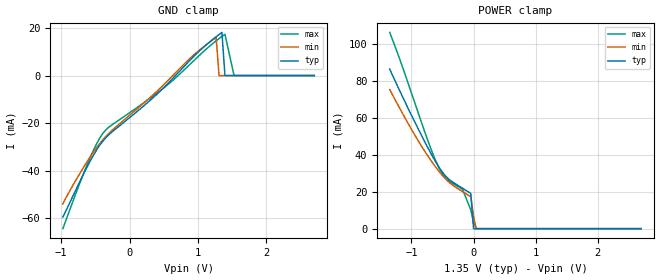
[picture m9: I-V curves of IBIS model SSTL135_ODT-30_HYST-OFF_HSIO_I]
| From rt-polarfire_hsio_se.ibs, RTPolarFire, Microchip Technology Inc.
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|   Model SSTL135_ODT-30_HYST-OFF_HSIO_I
[Model]   SSTL135_ODT-30_HYST-OFF_HSIO_I
Model_type   Input
Vinl =   0.585
Vinh =   0.765
|   typ   min   max
C_comp_pullup   1.335e-12   1.335e-12   1.380e-12
C_comp_pulldown  1.335e-12   1.335e-12   1.380e-12
[Temperature Range]  25C   125C   -55C
[Voltage Range]  1.35   1.2825   1.4175
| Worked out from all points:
|   POWER clamp passes 1 mA (typ) near -0.00 V on its own axis
[GND Clamp]
| Voltage   I(typ)   I(min)   I(max)
-974.5mV  -59.47mA   -53.9mA    -64.32mA
-575.9mV  -35.95mA   -34.19mA   -34.49mA
-443mV    -29.6mA    -28.82mA   -26.65mA
-354.4mV  -26.35mA   -25.8mA    -23.04mA
506.2mV   -4.877mA   -3.654mA   -5.045mA
928.1mV   7.72mA     8.419mA    5.967mA
1.266V    16.29mA    16.02mA    14.6mA
1.308V    17.22mA    0A         15.53mA
1.35V     18.14mA    0A         16.43mA
1.394V    0A         0A         17.36mA
1.527V    0A         0A         0A
2.7V      0A         0A         0A
[POWER Clamp]
| Voltage   I(typ)   I(min)   I(max)
-1.35V    86.58mA    75.43mA    106.5mA
-1.196V   75.3mA     65.72mA    92.61mA
-930.2mV  56.74mA    49.83mA    66.68mA
-708.7mV  42.18mA    38.09mA    45.29mA
-575.9mV  34.37mA    31.92mA    34.3mA
-487.3mV  30.02mA    28.3mA     28.99mA
-443mV    28.26mA    26.7mA     27.21mA
-177.2mV  21.9mA     20.1mA     21.43mA
-44.3mV   19.09mA    17.31mA    10.2mA
0V        0A         6.764mA    3.506mA
42.19mV   0A         0A         0A
2.7V      0A         0A         0A
